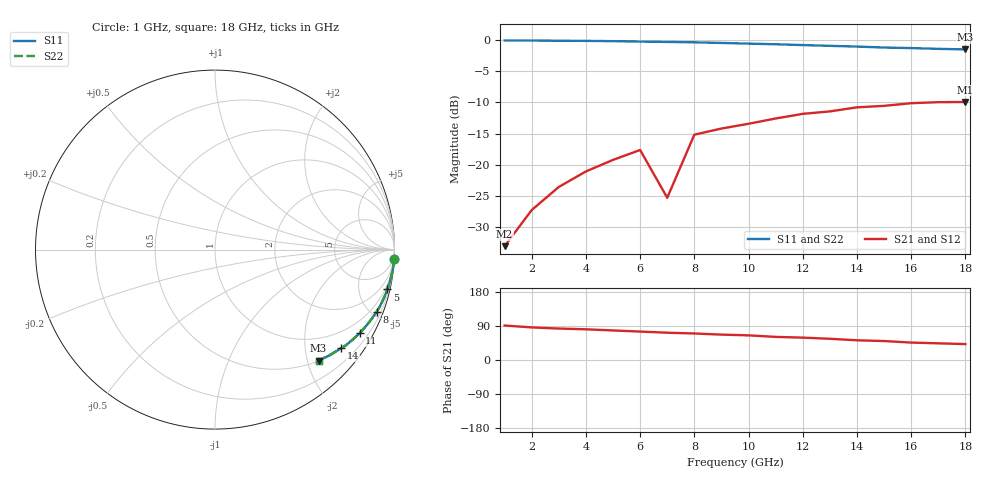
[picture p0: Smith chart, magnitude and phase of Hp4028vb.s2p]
!HPND-4028 beam lead PIN diode
!Series configuration S-parameters Vr= 10 V.  Last updated 10/3/97
# mhz s ma r 50
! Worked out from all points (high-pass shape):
!   18 points, 1 GHz to 18 GHz, reference 50 ohm
!   highest |S21| = -9.92 dB at 18 GHz (marker M1); lowest = -33.2 dB at 1 GHz (marker M2)
!   |S21| within 3 dB of the highest: 10.6 GHz to end of sweep
!   lowest |S11| = -1.5 dB at 18 GHz (marker M3), VSWR 11.99, Z = 25.3 - j110 ohm
!   |S11| at or under -10 dB: nowhere
!   |S22| runs from -1.5 to 0.0 dB; largest |S21 - S12| = 0
!   S11 on the Smith chart (normalised r, x): 1 GHz: 1, -38; 5 GHz: 0.55, -8.74; 8 GHz: 0.53, -5.34; 11 GHz: 0.52, -3.66; 14 GHz: 0.52, -2.82; 18 GHz: 0.51, -2.20
1000  0.999 -3.0  0.022 91.0  0.022 91.0  0.999 -3.0
2000  0.997 -6.0  0.043 86.0  0.043 86.0  0.997 -6.0
3000  0.994 -8.0  0.066 83.0  0.066 83.0  0.994 -8.0
4000  0.991 -10.0  0.088 81.0  0.088 81.0  0.991 -10.0
5000  0.986 -13.0  0.109 78.0  0.109 78.0  0.986 -13.0
6000  0.979 -16.0  0.131 75.0  0.131 75.0  0.979 -16.0
7000  0.972 -19.0  0.054 72.0  0.054 72.0  0.972 -19.0
8000  0.965 -21.0  0.174 70.0  0.174 70.0  0.965 -21.0
9000  0.954 -24.0  0.195 67.0  0.195 67.0  0.954 -24.0
10000  0.942 -27.0  0.213 65.0  0.213 65.0  0.942 -27.0
11000  0.931 -30.0  0.235 61.0  0.235 61.0  0.931 -30.0
12000  0.917 -33.0  0.256 59.0  0.256 59.0  0.917 -33.0
13000  0.904 -36.0  0.268 56.0  0.268 56.0  0.904 -36.0
14000  0.892 -38.0  0.289 52.0  0.289 52.0  0.892 -38.0
15000  0.876 -41.0  0.297 50.0  0.297 50.0  0.876 -41.0
16000  0.867 -43.0  0.312 46.0  0.312 46.0  0.867 -43.0
17000  0.855 -45.0  0.318 44.0  0.318 44.0  0.855 -45.0
18000  0.846 -47.0  0.319 42.0  0.319 42.0  0.846 -47.0
